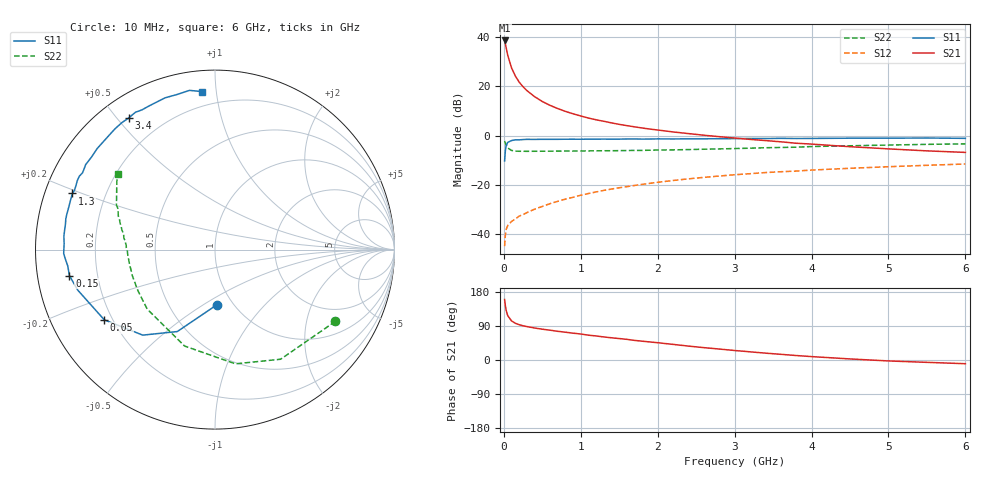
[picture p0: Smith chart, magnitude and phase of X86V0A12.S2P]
! SIEMENS Small Signal Semiconductors
! BFP136W
! Si NPN RF Bipolar Junction Transistor in SOT343
! VCE = 6 V  IC = 120 mA
! Common Emitter S-Parameters:  September  1994
# GHz  S  MA  R  50
!  f  S11  S21  S12  S22
! GHz  MAG  ANG  MAG  ANG  MAG  ANG  MAG  ANG
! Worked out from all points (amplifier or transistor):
!   40 points, 10 MHz to 6 GHz, reference 50 ohm
!   highest |S21| = 38.7 dB at 10 MHz (marker M1)
!   |S21| within 3 dB of that: start of sweep to 30.39 MHz
!   unconditionally stable (mu >= 1): 563.7 MHz to 3.024 GHz
!   at 200 MHz: K = 0.69, MSG = 27.2 dB, |S12| = -32.7 dB
!   at 1.5 GHz: K = 1.11, MAG = 10.9 dB, |S12| = -21.1 dB
!   at 6 GHz: K = 0.97, MSG = 2.4 dB, |S12| = -11.5 dB
!   S11 on the Smith chart (normalised r, x): 10 MHz: 0.84, -0.57; 50 MHz: 0.17, -0.28; 150 MHz: 0.10, -0.09; 1.3 GHz: 0.08, +0.19; 3.4 GHz: 0.08, +0.54; 6 GHz: 0.11, +0.91
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0.01  0.3076 -88.0  86.14 159.7  0.0057 68.9  0.7808 -30.8
0.02  0.5025 -114.7  73.27 143.0  0.0095 56.7  0.7119 -59.1
0.03  0.6239 -130.2  61.39 131.1  0.0124 48.8  0.6464 -79.9
0.05  0.7304 -147.6  43.5 117.2  0.0149 39.4  0.5634 -107.5
0.1  0.7977 -163.6  23.91 103.1  0.0181 37.7  0.5025 -138.7
0.15  0.824 -169.9  16.26 96.9  0.0204 39.8  0.4869 -151.6
0.2  0.8252 -173.6  12.22 93.1  0.0233 42.1  0.4827 -158.5
0.25  0.8357 -176.5  9.862 90.3  0.025 44.4  0.4831 -163.0
0.3  0.8433 -178.5  8.245 88.2  0.0274 46.5  0.4815 -166.0
0.4  0.8412 177.7  6.213 84.4  0.0322 50.1  0.483 -170.1
0.5  0.8452 175.0  4.955 81.3  0.0366 53.2  0.4839 -172.9
0.6  0.8448 172.7  4.134 78.7  0.0416 55.2  0.4849 -174.7
0.7  0.8452 170.3  3.565 75.7  0.0465 57.1  0.4863 -176.0
0.9  0.8489 166.6  2.789 70.8  0.0561 58.4  0.4881 -178.7
1.1  0.8496 162.2  2.282 65.5  0.0669 59.3  0.4916 179.7
1.3  0.8535 158.5  1.962 60.8  0.0775 59.5  0.4948 177.9
2.2  0.8597 143.2  1.193 41.2  0.123 54.1  0.5149 171.1
3.2  0.8773 126.3  0.842 21.6  0.1691 45.1  0.5573 162.6
3.4  0.8769 123.3  0.797 18.1  0.1784 43.0  0.57 160.9
4.5  0.8901 108.2  0.598 2.8  0.2178 33.7  0.6244 151.4
5.5  0.8984 99.1  0.492 -6.2  0.2504 25.6  0.6674 145.0
6  0.8834 94.7  0.458 -9.8  0.2664 21.2  0.6828 142.0
